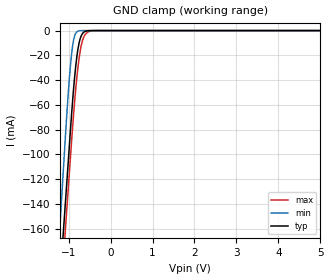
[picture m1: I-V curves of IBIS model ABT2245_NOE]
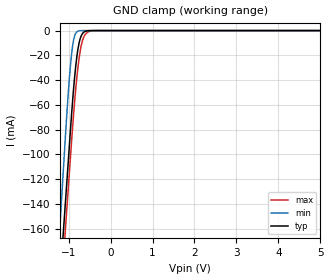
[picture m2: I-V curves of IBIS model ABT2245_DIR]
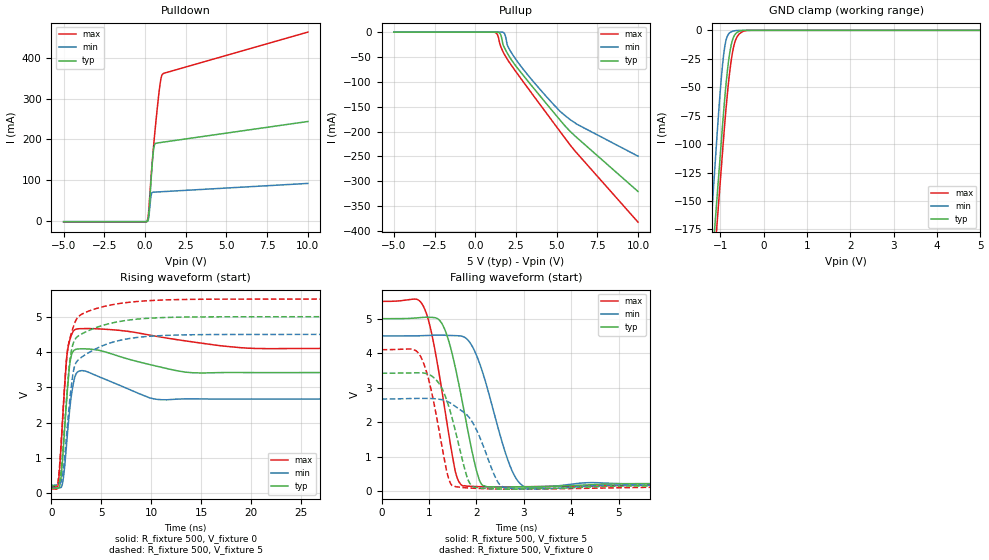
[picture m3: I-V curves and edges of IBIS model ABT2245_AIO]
| TEXAS INSTRUMENTS INCORPORATED
| Standard Linear and Logic Group
| IBIS Model of SN74ABT2245
| OCTAL TRANSCEIVERS AND LINE/MOS DRIVERS WITH 3-STATE OUTPUTS
| This file contains package information for the following:
|  SOIC 20-pin (DW) package as [Component] ABT2245_DW
|  SSOP 20-pin (DB) package as [Component] ABT2245_DB
|  P-DIP 20-pin (N) package as [Component] ABT2245_N
|  TSSOP 20-pin (PW) package as [Component] ABT2245_PW
| This device can be powered at the following Vccs:
|  5 volt Vcc
| This file provides unique models under the [Model Selector] for each Vcc.
| For operation at a specific Vcc, select the appropriate model after each
| [Model Selector] keyword.
[IBIS Ver]   3.2
[Comment char]  |_char
[File Name]   sn74abt2245.ibs
[File Rev]   1.2 | f_die
[Date]   September 15,2004
[Source]   Data created from TI-SPICE simulations at TI-SLL.
[Notes]   The following is an IBIS list for the ABT2245.
   Please contact sllibis@ti.com with questions and
   comments concerning SLL IBIS models.
   - FILE REV HISTORY
   - 1.2 Re-Release IBIS file on 09/17/04
   - Power clamp data deleted as there is no power-clamp diode.
   This IBIS model is created from a BA (back annotated netlist
   Non-Convergence in the following files:
   - pu_abt2245_aio_50, extrapolated from 7.065 V plus
   - pu_abt2245_bio_50, extrapolated from ~7 V plus
[Disclaimer] Property of Texas Instruments Incorporated.  Unauthorized
   reproduction and/or distribution is strictly prohibited.
   This product is protected under copyright law.
   Created  2001, (C) Copyright  2001, Texas Instruments
   Incorporated, All Rights Reserved
   UNLESS THERE IS A SIGNED, WRITTEN AGREEMENT TO THE
   CONTRARY, TEXAS INSTRUMENTS (TI) IS PROVIDING THE IBIS
   MODELS  AND WITHOUT ANY WARRANTY, EXPRESSED OR
   IMPLIED.  TI assumes no liability for:
   1) the accuracy of the IBIS models provided to your
   company;
   2) the proper functioning of these IBIS Models in your
   design or for any resulting applications; or
   3) infringement of patents, copyrights or intellectual
   property rights resulting from your use of these IBIS
   models.
   TI provides IBIS Models as a service to our customers.
   You and your company shall not distribute, sell or give
   these models to anyone else without prior written
   permission from TI.
   TI reserves the right to make changes to our products or
   to discontinue any semiconductor product or service
   without notice, and advises our customers to obtain the
   latest version of relevant information to verify, before
   placing orders, that the information being relied on is
   current.
   Please be aware that your receipt and use of the IBIS
   information provided shall serve as acceptance of these
   terms and conditions.  If you do not accept these terms,
   you should return or destroy the IBIS models and any
   other accompanying information immediately.
| Component ABT2245_DW 20-pin SOIC
[Component]   ABT2245_DW
[Manufacturer]   Texas Instruments, Inc.
[Package]
|   typ   min   max
R_pkg   3.800e-02   3.300e-02   4.500e-02
L_pkg   5.012e-09   4.110e-09   6.349e-09
C_pkg   7.170e-13   5.300e-13   8.680e-13
[Pin]   signal_name   model_name   R_pin   L_pin   C_pin
1   DIR   ABT2245_DIR   4.200e-02   6.336e-09   8.650e-13
2   A1   ABT2245_AIO   4.300e-02   5.542e-09   8.670e-13
3   A2   ABT2245_AIO   3.400e-02   4.714e-09   7.320e-13
4   A3   ABT2245_AIO   3.400e-02   4.377e-09   5.910e-13
5   A4   ABT2245_AIO   3.600e-02   4.130e-09   5.330e-13
6   A5   ABT2245_AIO   3.500e-02   4.111e-09   5.300e-13
7   A6   ABT2245_AIO   3.400e-02   4.284e-09   5.830e-13
8   A7   ABT2245_AIO   3.400e-02   4.634e-09   7.260e-13
9   A8   ABT2245_AIO   4.000e-02   5.518e-09   8.650e-13
10   GND   GND   4.300e-02   6.349e-09   8.660e-13
11   B8   ABT2245_BIO   4.100e-02   6.281e-09   8.610e-13
12   B7   ABT2245_BIO   4.500e-02   5.561e-09   8.680e-13
13   B6   ABT2245_BIO   3.300e-02   4.778e-09   7.420e-13
14   B5   ABT2245_BIO   3.500e-02   4.414e-09   5.960e-13
15   B4   ABT2245_BIO   3.500e-02   4.110e-09   5.330e-13
16   B3   ABT2245_BIO   3.600e-02   4.130e-09   5.330e-13
17   B2   ABT2245_BIO   3.400e-02   4.377e-09   5.910e-13
18   B1   ABT2245_BIO   3.400e-02   4.714e-09   7.310e-13
19   NOE   ABT2245_NOE   4.300e-02   5.569e-09   8.680e-13
20   VCC   POWER   4.200e-02   6.308e-09   8.640e-13
| Component ABT2245_DB 20-pin
[Component]   ABT2245_DB
[Manufacturer]   Texas   Instruments,   Inc.
[Package]
|   Mean.   Min.   Max.
R_pkg   0.04   0.035   0.051
L_pkg   3.495nH  3.035nH   4.314nH
C_pkg   0.42pF   0.346pF   0.502pF
[Pin]   signal_name   model_name   R_pin   L_pin   C_pin
1   DIR   ABT2245_DIR   0.049   4.31nH   0.502pF
2   A1   ABT2245_AIO   0.048   3.903nH   0.487pF
3   A2   ABT2245_AIO   0.035   3.189nH   0.396pF
4   A3   ABT2245_AIO   0.035   3.036nH   0.347pF
5   A4   ABT2245_AIO   0.035   3.035nH   0.367pF
6   A5   ABT2245_AIO   0.035   3.035nH   0.367pF
7   A6   ABT2245_AIO   0.035   3.036nH   0.347pF
8   A7   ABT2245_AIO   0.035   3.189nH   0.397pF
9   A8   ABT2245_AIO   0.047   3.899nH   0.488pF
10   GND   GND   0.051   4.314nH   0.5pF
11   B8   ABT2245_BIO   0.051   4.314nH   0.5pF
12   B7   ABT2245_BIO   0.047   3.899nH   0.488pF
13   B6   ABT2245_BIO   0.035   3.189nH   0.397pF
14   B5   ABT2245_BIO   0.035   3.036nH   0.346pF
15   B4   ABT2245_BIO   0.035   3.035nH   0.367pF
16   B3   ABT2245_BIO   0.035   3.035nH   0.367pF
17   B2   ABT2245_BIO   0.035   3.036nH   0.346pF
18   B1   ABT2245_BIO   0.035   3.189nH   0.397pF
19   OEN   ABT2245_NOE   0.047   3.899nH   0.488pF
20   VCC   POWER   0.051   4.314nH   0.502pF
| Component ABT2245_N 20-pin
[Component]   ABT2245_N
[Manufacturer]   Texas   Instruments,   Inc.
[Package]
|   Mean.   Min.   Max.
R_pkg   0.043   0.038   0.05
L_pkg   7.384nH   4.68nH   10.321nH
C_pkg   0.51pF   0.231pF   0.821pF
[Pin]   signal_name   model_name   R_pin   L_pin   C_pin
1   DIR  ABT2245_DIR   0.042   9.427nH   0.81pF
2   A1   ABT2245_AIO   0.046   8.544nH   0.456pF
3   A2   ABT2245_AIO   0.048   7.163nH   0.435pF
4   A3   ABT2245_AIO   0.04   4.825nH   0.261pF
5   A4   ABT2245_AIO   0.04   5.284nH   0.648pF
6   A5   ABT2245_AIO   0.04   4.686nH   0.232pF
7   A6   ABT2245_AIO   0.04   6.359nH   0.489pF
8   A7   ABT2245_AIO   0.038   7.982nH   0.475pF
9   A8   ABT2245_AIO   0.043   9.403nH   0.475pF
10   GND  GND   0.05   10.321nH  0.805pF
11   B8   ABT2245_BIO   0.05   10.281nH  0.81pF
12   B7   ABT2245_BIO   0.043   9.383nH   0.477pF
13   B6   ABT2245_BIO   0.038   7.978nH   0.476pF
14   B5   ABT2245_BIO   0.04   6.302nH   0.492pF
15   B4   ABT2245_BIO   0.04   4.68nH   0.231pF
16   B3   ABT2245_BIO   0.04   5.284nH   0.648pF
17   B2   ABT2245_BIO   0.04   4.822nH   0.261pF
18   B1   ABT2245_BIO   0.047   7.118nH   0.439pF
19   OEN  ABT2245_NOE   0.046   8.492nH   0.461pF
20   VCC  POWER   0.043   9.348nH   0.821pF
| Component ABT2245_PW 20-pin TSSOP
[Component]   ABT2245_PW
[Manufacturer]   Texas Instruments, Inc.
[Package]
|   typ   min   max
R_pkg   5.000e-02   4.200e-02   6.000e-02
L_pkg   2.802e-09   2.248e-09   3.553e-09
C_pkg   3.170e-13   2.020e-13   4.430e-13
[Pin]   signal_name   model_name   R_pin   L_pin   C_pin
1   DIR   ABT2245_DIR   5.500e-02   3.461e-09   4.400e-13
2   A1   ABT2245_AIO   5.500e-02   3.150e-09   4.010e-13
3   A2   ABT2245_AIO   4.200e-02   2.619e-09   3.020e-13
4   A3   ABT2245_AIO   4.500e-02   2.273e-09   2.020e-13
5   A4   ABT2245_AIO   4.500e-02   2.248e-09   2.240e-13
6   A5   ABT2245_AIO   4.500e-02   2.273e-09   2.260e-13
7   A6   ABT2245_AIO   4.400e-02   2.323e-09   2.050e-13
8   A7   ABT2245_AIO   4.600e-02   2.704e-09   3.070e-13
9   A8   ABT2245_AIO   6.000e-02   3.265e-09   4.110e-13
10   GND   GND   5.700e-02   3.506e-09   4.360e-13
11   B8   ABT2245_BIO   5.800e-02   3.553e-09   4.370e-13
12   B7   ABT2245_BIO   5.800e-02   3.193e-09   4.050e-13
13   B6   ABT2245_BIO   4.200e-02   2.704e-09   3.110e-13
14   B5   ABT2245_BIO   4.600e-02   2.392e-09   2.100e-13
15   B4   ABT2245_BIO   4.700e-02   2.334e-09   2.290e-13
16   B3   ABT2245_BIO   4.700e-02   2.300e-09   2.270e-13
17   B2   ABT2245_BIO   4.700e-02   2.349e-09   2.070e-13
18   B1   ABT2245_BIO   4.500e-02   2.677e-09   3.060e-13
19   OEN   ABT2245_NOE   6.000e-02   3.235e-09   4.060e-13
20   VCC   POWER   5.600e-02   3.487e-09   4.430e-13
| Models and submodels in the file (4): ABT2245_NOE (Input), ABT2245_DIR (Input), ABT2245_AIO (I/O), ABT2245_BIO (I/O)
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[Model]   ABT2245_NOE
Model_type  Input
Vinl=0.8
Vinh=2.0
| variable   typ   min   max
C_comp   3.05pF   2.39pF   4.54pF
[Temperature Range]   40   -40   100
| Ambient temperature   25   -40   85
[Voltage range]   5   4.5   5.5
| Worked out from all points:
|   GND clamp passes 1 mA (typ) near -0.62 V on its own axis
[GND Clamp]
| ABT2245_NOE
|   Voltage   I(typ)   I(min)   I(max)
-5V       -2.087A    -2.3A      -2.099A
-1.215V   -207.8mA   -163.2mA   -229.9mA
-1.12V    -160.8mA   -110.4mA   -182.8mA
-1.075V   -138.9mA   -85.43mA   -160.5mA
-1V       -102.4mA   -47.35mA   -124.1mA
-925mV    -66.35mA   -18.07mA   -87.99mA
-850mV    -35.87mA   -3.783mA   -55.41mA
-775mV    -14.74mA   -473.3uA   -29.52mA
-725mV    -6.765mA   -69.07uA   -17.06mA
-650mV    -1.717mA   -1.985uA   -6.254mA
-450mV    -7.801uA   -255.5pA   -218.6uA
5V        31.82pA    20.18pA    989.6pA
[Model]   ABT2245_DIR
Model_type  Input
Vinl=0.8
Vinh=2.0
| variable   typ   min   max
C_comp   3.09pF   2.43pF   4.57pF
[Temperature Range]   40   -40   100
| Ambient temperature   25   -40   85
[Voltage range]   5   4.5   5.5
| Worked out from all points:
|   GND clamp passes 1 mA (typ) near -0.62 V on its own axis
[GND Clamp]
| ABT2245_DIR
|   Voltage   I(typ)   I(min)   I(max)
-5V       -2.087A    -2.3A      -2.099A
-1.215V   -207.8mA   -163.2mA   -229.9mA
-1.12V    -160.8mA   -110.4mA   -182.8mA
-1.075V   -138.9mA   -85.43mA   -160.5mA
-1V       -102.4mA   -47.35mA   -124.1mA
-925mV    -66.35mA   -18.07mA   -87.99mA
-850mV    -35.87mA   -3.783mA   -55.41mA
-775mV    -14.74mA   -473.3uA   -29.52mA
-725mV    -6.765mA   -69.07uA   -17.06mA
-650mV    -1.717mA   -1.985uA   -6.254mA
-450mV    -7.801uA   -255.5pA   -218.6uA
5V        31.82pA    20.18pA    989.6pA
[Model]   ABT2245_AIO
Model_type  I/O
Vinl=0.8
Vinh=2.0
Enable   Active-Low
Vref =   0
Rref =   500
Cref =   50p
Vmeas =   1.5
| variable   typ   min   max
C_comp   6.13pF   4.91pF   8.69pF
| C_pullup   5.61pF   0.41pF   8.76pF
| C_pulldown   7.55pF   0.55pF   25.00pF
| C_tri-state   6.13pF   4.91pF   8.69pF
[Temperature Range]   40   -40   100
| Ambient temperature   25   -40   85
[Voltage range]   5   4.5   5.5
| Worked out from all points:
|   slope of the pulldown table from 0 to 0.75 V, typ, clamps not added: 3.88 ohm
|   GND clamp passes 1 mA (typ) near -0.57 V on its own axis
|   rising waveform, R_fixture 500, V_fixture 0: 20-80 % time 483ps typ, 466ps min, 515ps max; typ from 0.15 V to 3.42 V
|   falling waveform, R_fixture 500, V_fixture 5: 20-80 % time 429ps typ, 537ps min, 389ps max; typ from 5 V to 0.214 V
|   rising waveform, R_fixture 500, V_fixture 5: 20-80 % time 875ps typ, 1.03ns min, 964ps max; typ from 0.214 V to 5 V
|   falling waveform, R_fixture 500, V_fixture 0: 20-80 % time 383ps typ, 493ps min, 346ps max; typ from 3.42 V to 0.15 V
[GND Clamp]
| ABT2245_AIO
|   Voltage   I(typ)   I(min)   I(max)
-5V       -2.728A    -2.793A    -2.802A
-1.25V    -234.3mA   -190mA     -260mA
-1.2V     -208.6mA   -161.4mA   -233.5mA
-1.14V    -177.8mA   -127.3mA   -202.2mA
-1.075V   -145.2mA   -90.34mA   -168.6mA
-975mV    -95.27mA   -39.93mA   -118.5mA
-900mV    -59.46mA   -14.28mA   -81.91mA
-825mV    -30.71mA   -3.897mA   -50.12mA
-750mV    -12.53mA   -1.277mA   -26.18mA
-625mV    -2.093mA   -103.7uA   -6.308mA
-400mV    -7.633uA   -3.482nA   -174uA
5V        82.8pA     75.18pA    1.574nA
[Pulldown]
| ABT2245_AIO
|   Voltage   I(typ)   I(min)   I(max)
-5V       -2.416mA   -1.725mA   -3.213mA
115mV     -1.623mA   -1.411mA   -1.085mA
170mV     1.291mA    -186.2uA   5.424mA
230mV     15.79mA    9.416mA    26.89mA
385mV     108.3mA    64.29mA    114.5mA
480mV     157.8mA    70.2mA     161.9mA
555mV     181.9mA    70.46mA    196.3mA
635mV     189.6mA    70.65mA    230.1mA
915mV     191.9mA    71.28mA    332.8mA
1.005V    192.4mA    71.49mA    353.3mA
1.105V    193mA      71.71mA    360.8mA
10V       243.7mA    91.85mA    462.9mA
[Pullup]
| ABT2245_AIO
|   Voltage   I(typ)   I(min)   I(max)
-5V       -7.129pA   -6.201pA   -14.2pA
1.275V    -34.88uA   -8.423nA   -1.495mA
1.395V    -305.5uA   -207nA     -7.72mA
1.545V    -3.959mA   -8.606uA   -27.03mA
1.78V     -30.49mA   -2.055mA   -44.05mA
1.86V     -35.67mA   -8.553mA   -48.75mA
2.005V    -44.26mA   -28.66mA   -56.41mA
2.595V    -72.38mA   -59.54mA   -83.97mA
3.875V    -124.2mA   -111.2mA   -141mA
5.195V    -176.4mA   -158.8mA   -199.2mA
6.21V     -211.3mA   -184.7mA   -242.2mA
10V       -320.6mA   -249.6mA   -382.3mA
[Ramp]
| ABT2245_AIO
| variable   typ   min   max
dV/dt_r   2.37/6.03E-10   1.99/6.75E-10   2.73/6.07E-10
dV/dt_f   2.95/4.43E-10   2.64/5.60E-10   3.26/4.01E-10
R_load = 500
[Rising Waveform]
| ABT2245_AIO
R_fixture =   500
C_fixture =   0
L_fixture =   0
V_fixture =   0
V_fixture_min = 0
V_fixture_max = 0
|   Time   V(typ)   V(min)   V(max)
0s        149.8mV    166.5mV    126.1mV
655ps     143.4mV    153.8mV    224.8mV
880ps     270.7mV    157.7mV    941.1mV
1.095ns   871.6mV    257.9mV    1.954V
1.62ns    2.986V     1.724V     4.044V
1.965ns   3.863V     2.696V     4.448V
2.49ns    4.079V     3.391V     4.648V
11.05ns   3.566V     2.65V      4.419V
20.46ns   3.418V     2.67V      4.101V
49.99ns   3.419V     2.671V     4.101V
[Falling Waveform]
| ABT2245_AIO
R_fixture =   500
C_fixture =   0
L_fixture =   0
V_fixture =   5
V_fixture_min = 4.5
V_fixture_max = 5.5
|   Time   V(typ)   V(min)   V(max)
0s        4.999V     4.499V     5.499V
905ps     5.038V     4.508V     5.291V
1.08ns    5.033V     4.518V     4.415V
1.325ns   4.715V     4.519V     2.459V
1.555ns   3.592V     4.507V     581.4mV
1.725ns   2.439V     4.476V     154.3mV
2.11ns    202.1mV    3.539V     132.9mV
2.705ns   122.5mV    756.4mV    129.3mV
3.075ns   130mV      111.3mV    133.1mV
49.99ns   213.6mV    226.9mV    191.5mV
[Rising Waveform]
| ABT2245_AIO
R_fixture =   500
C_fixture =   0
L_fixture =   0
V_fixture =   5
V_fixture_min = 4.5
V_fixture_max = 5.5
|   Time   V(typ)   V(min)   V(max)
0s        213.7mV    226.8mV    191.6mV
600ps     231mV      241.2mV    244.4mV
880ps     431.8mV    293mV      1.016V
1.145ns   1.216V     560.5mV    2.224V
1.475ns   2.518V     1.492V     3.656V
1.74ns    3.455V     2.349V     4.258V
2.345ns   4.347V     3.618V     4.829V
3.72ns    4.607V     3.98V      5.158V
11.29ns   4.977V     4.47V      5.475V
49.99ns   4.999V     4.499V     5.499V
[Falling Waveform]
| ABT2245_AIO
R_fixture =   500
C_fixture =   0
L_fixture =   0
V_fixture =   0
V_fixture_min = 0
V_fixture_max = 0
|   Time   V(typ)   V(min)   V(max)
0s        3.419V     2.671V     4.101V
780ps     3.431V     2.69V      3.998V
970ps     3.399V     2.689V     3.355V
1.175ns   3.189V     2.673V     2.051V
1.445ns   2.332V     2.561V     256.2mV
1.81ns    381.8mV    2.198V     97.88mV
1.945ns   125.5mV    1.934V     88.49mV
2.465ns   66.56mV    244.1mV    64.4mV
2.905ns   66.47mV    73.87mV    62.95mV
49.99ns   149.8mV    166.6mV    126.1mV
